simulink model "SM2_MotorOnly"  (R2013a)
settings: Solver=ode45  StartTime=0  StopTime=2  FixedStep=1e-4  RelTol=1e-3  AbsTol=1e-4
PreLoadFcn:
  | warning('off','sm:sli:setup:compile:LocalSolverNotSupported')
InitFcn:
  | if(~Model.ModelUpdate)
  |  [~]=SM2_MotorOnly_ConstrFnc(0,Model);
  | SimParam.IC = SM2_InitCondConstrFnc(RawParam,IC);
  |  Model.ModelUpdate=1;
  | end
model workspace (MAT data in the model file):
  handle : class17 (value not decoded)
  handle : class17 (value not decoded)
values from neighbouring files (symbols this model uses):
  RawParam = RobotParamGather(ParamLib)    [DeltaModelMain_v2.m]    (also in main_TimeSimulation.m; MGI.m = y)
libraries: SM2_MotorPartsLib x1, SM2_FramePartsLib x1

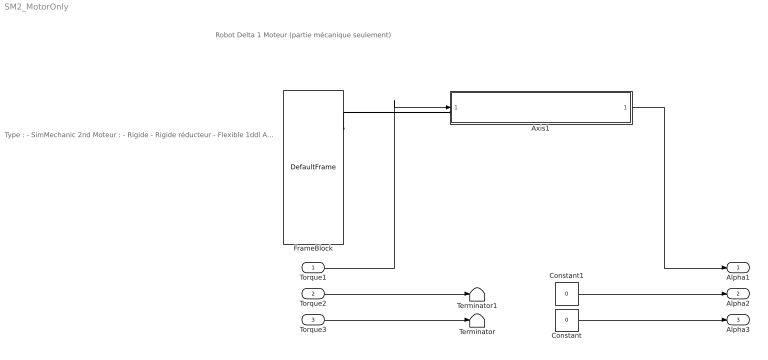
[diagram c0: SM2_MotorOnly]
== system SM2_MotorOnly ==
  note: Robot Delta 1 Moteur (partie mécanique seulement)
  note: Type : - SimMechanic 2nd Moteur : - Rigide - Rigide réducteur - Flexible 1ddl Avec Volant d'inertie rigide
  Torque1 : Inport
  Torque2 : Inport  Port=2
  Torque3 : Inport  Port=3
  Axis1 : Subsystem
  Constant : Constant  Value=0
  Constant1 : Constant  Value=0
  FrameBlock : SM2_FramePartsLib/DefaultFrame
  Terminator : Terminator
  Terminator1 : Terminator
  Alpha1 : Outport
  Alpha2 : Outport  Port=2
  Alpha3 : Outport  Port=3
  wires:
  Axis1/1(Alpha) -> Alpha1/1
  Constant/1 -> Alpha3/1
  Torque3/1 -> Terminator/1
  Torque2/1 -> Terminator1/1
  Constant1/1 -> Alpha2/1
  Torque1/1 -> Axis1/1(Torque)
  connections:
  FrameBlock/RConn1 -- Axis1/LConn1

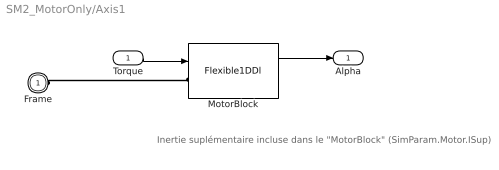
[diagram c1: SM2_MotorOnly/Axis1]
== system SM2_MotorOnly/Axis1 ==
  note: Inertie suplémentaire incluse dans le "MotorBlock" (SimParam.Motor.ISup)
  Torque : Inport
  MotorBlock : SM2_MotorPartsLib/Flexible1DDl  VariantControl=motorVarFlex1
  Frame : PMIOPort  Port=1  Side=Left
  Alpha : Outport
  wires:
  MotorBlock/1 -> Alpha/1
  Torque/1 -> MotorBlock/1
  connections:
  Frame/RConn1 -- MotorBlock/LConn1
